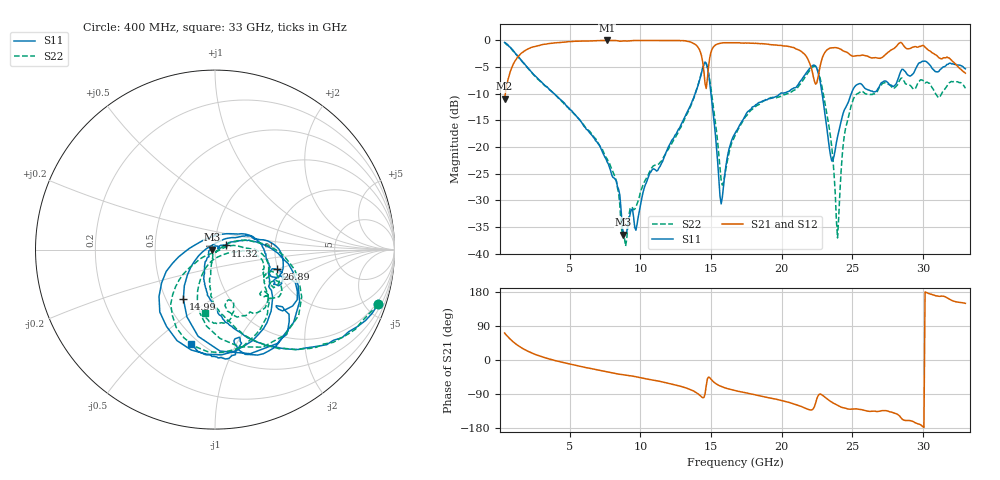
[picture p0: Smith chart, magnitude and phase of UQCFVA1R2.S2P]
!  Part Number  UQCFVA1R2  Mounting Orientation: Horizontal
!  Description: Ultra Low ESR Microwave capacitors
!  Application: Coupling, Bypass, Tuning, DC Block
!  Filters, Matching
# GHZ S DB R 50
! Freq  |S11|  S11 Ph  |S21|  S21 Ph  |S12|  S12 Ph  |S22|  S22 Ph
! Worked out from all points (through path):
!   401 points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, 400 MHz to 33 GHz, reference 50 ohm
!   highest |S21| = 0.00 dB at 7.654 GHz (marker M1); lowest = -10.9 dB at 400 MHz (marker M2)
!   group delay of S21, straight-line fit = 18.4 ps
!   lowest |S11| = -36.4 dB at 8.795 GHz (marker M3), VSWR 1.03, Z = 48.5 + j0.0177 ohm
!   |S11| at or under -10 dB: 3.914 GHz to 13.88 GHz (9.968 GHz wide, 112 % of centre); 15 GHz to 19.9 GHz (4.901 GHz wide, 28.1 % of centre); 22.86 GHz to 24.92 GHz (2.06 GHz wide, 8.62 % of centre)
!   |S22| runs from -38.6 to -0.4 dB; largest |S21 - S12| = 0.013
!   S11 on the Smith chart (normalised r, x): 400 MHz: 0.80, -6.01; 11.32 GHz: 1.12, +0.05; 14.99 GHz: 0.61, -0.38; 26.89 GHz: 1.98, -0.50; 33 GHz: 0.45, -0.67
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0.4  -0.37 -18.6  -10.94 71.3  -10.94 71.3  -0.36 -18.6
2.356  -6.09 -71.9  -1.25 17.9  -1.29 17.5  -6.14 -71.9
5.861  -15.43 -111.6  -0.11 -17.7  -0.11 -17.8  -15.40 -100.3
7.654  -22.79 -129.8  0.00 -31.1  -0.01 -31.3  -22.22 -103.9
8.795  -36.41 179.3  -0.09 -38.8  -0.09 -38.8  -35.81 -73.8
11.321  -23.91 21.4  -0.01 -55.9  -0.01 -55.9  -23.14 20.6
14.337  -5.96 -23.1  -2.95 -97.5  -2.97 -97.4  -6.01 -20.6
14.663  -4.26 -71.3  -9.02 -68.2  -8.83 -68.3  -4.36 -63.9
14.989  -9.72 -122.7  -2.32 -49.9  -2.37 -50.3  -8.78 -103.3
15.722  -30.67 121.4  -0.50 -69.7  -0.52 -69.8  -26.31 -88.0
16.7  -17.46 30.1  -0.41 -80.5  -0.43 -80.6  -17.85 -5.4
20.449  -9.59 -24.8  -1.10 -111.0  -1.17 -111.0  -9.98 -30.7
22.161  -4.76 -79.8  -5.77 -131.2  -5.78 -131.3  -5.01 -74.0
22.731  -7.81 -140.0  -4.74 -89.8  -4.73 -90.4  -7.18 -122.8
23.465  -21.68 139.5  -1.41 -109.3  -1.44 -109.6  -18.21 -146.5
23.954  -18.11 45.3  -1.41 -119.5  -1.40 -119.8  -37.06 -63.5
24.443  -12.98 18.6  -2.06 -126.6  -2.09 -126.7  -17.66 8.5
25.013  -9.40 3.6  -2.93 -129.5  -2.93 -129.6  -11.45 -5.9
26.888  -8.78 -17.6  -3.33 -135.4  -3.37 -135.8  -8.89 -21.3
27.621  -8.33 -30.1  -2.06 -136.1  -2.01 -135.9  -8.26 -32.9
29.985  -3.90 -58.9  -0.92 -175.6  -0.97 -175.5  -7.48 -56.3
33  -5.32 -104.3  -6.14 149.5  -6.15 149.7  -8.98 -99.3
